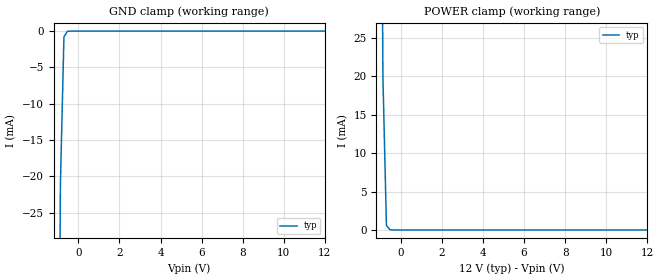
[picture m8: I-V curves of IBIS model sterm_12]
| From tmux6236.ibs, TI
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| sterm_12
[Model]   sterm_12
Model_type   Terminator
|   typ   min   max
C_comp   2.533030e-11   NA   NA
[Voltage Range]   12   NA   NA
[Temperature Range]   27   NA   NA
[Power Clamp Reference]   12   NA   NA
[GND Clamp Reference]   0   NA   NA
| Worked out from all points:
|   GND clamp passes 1 mA (typ) near -0.71 V on its own axis
|   POWER clamp passes 1 mA (typ) near -0.71 V on its own axis
[GND Clamp]
|   Voltage   I(typ)   I(min)   I(max)
-5V       -6.893A    NA         NA
-1.051V   -101.8mA   NA         NA
-878.8mV  -21.07mA   NA         NA
-707.1mV  -806uA     NA         NA
-535.4mV  -21.38uA   NA         NA
12V       5.313nA    NA         NA
[POWER Clamp]
|   Voltage   I(typ)   I(min)   I(max)
-5V       7.102A     NA         NA
-1.05V    98.01mA    NA         NA
-878.8mV  19.93mA    NA         NA
-707.1mV  596uA      NA         NA
-535.4mV  25.39uA    NA         NA
12V       -4.959nA   NA         NA
